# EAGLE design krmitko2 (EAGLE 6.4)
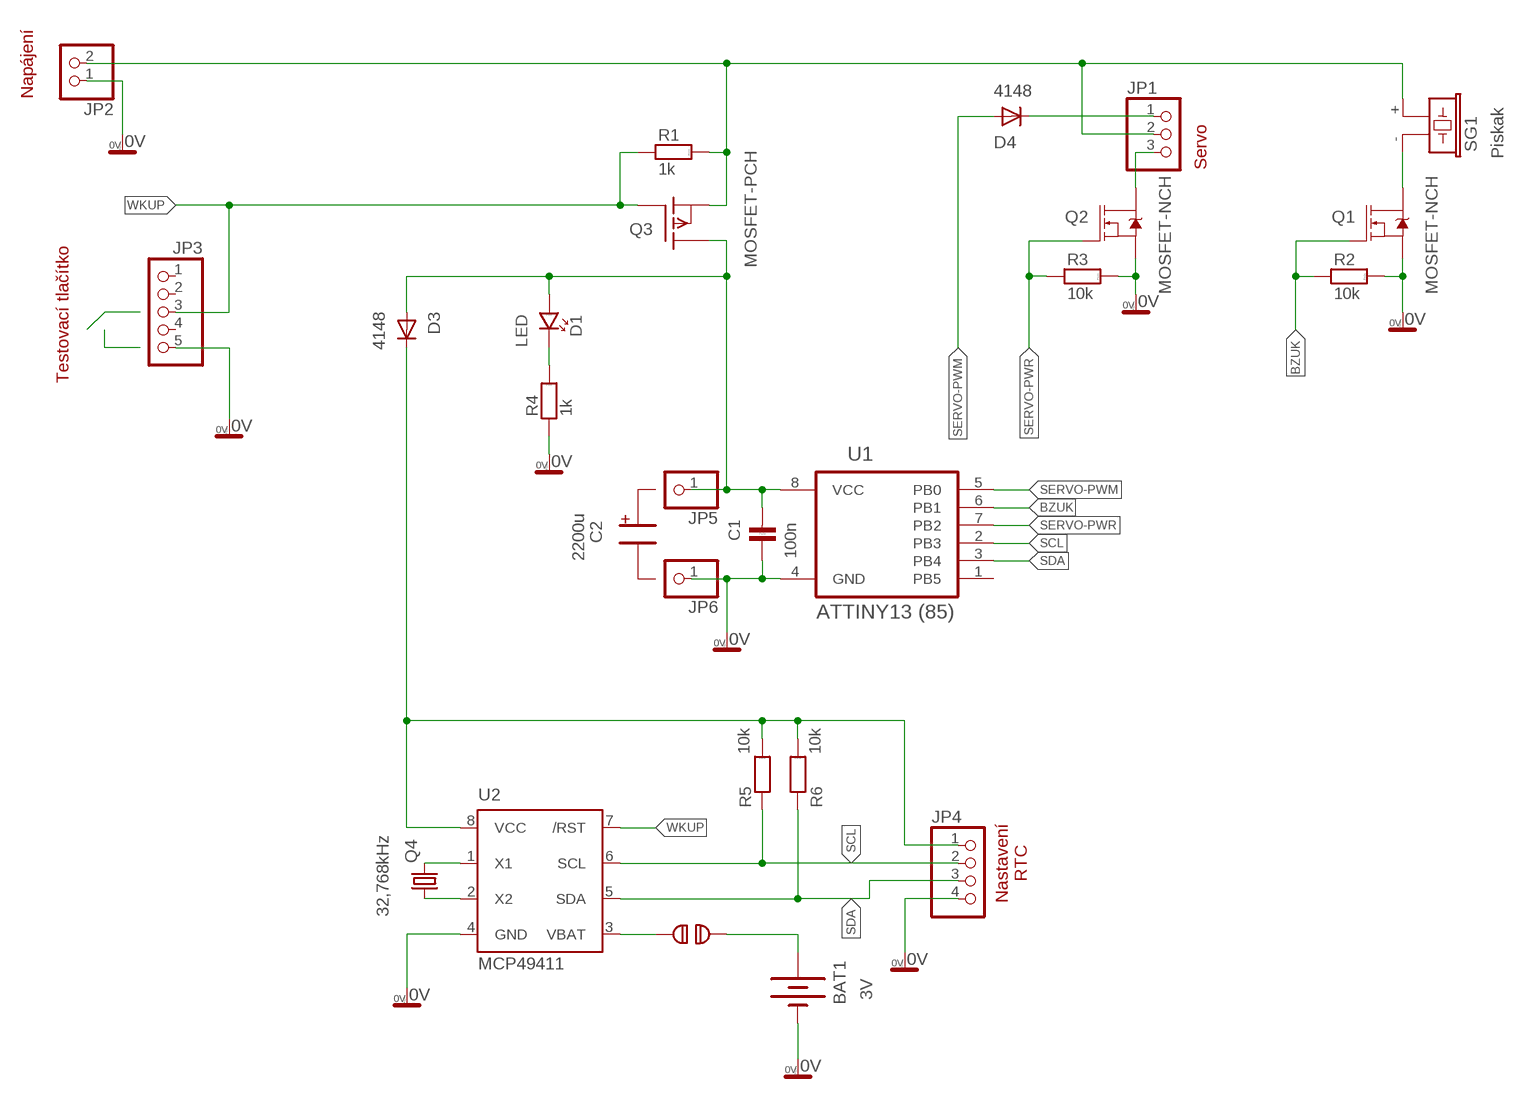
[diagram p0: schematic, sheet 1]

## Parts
BAT1  3V  BATTERY20PTH2  [BATTERY]
C1  100n  C-KER_0805  [0805]
D1  LED  LED_3  [LED_3]
D3  4148  CGRM4001-G  [SOD-123_MINI-SMA]
D4  4148  CGRM4001-G  [SOD-123_MINI-SMA]
JP1  PINHD-1X3  [1X03]
JP2  PINHD-1X2  [1X02]
JP3  PINHD-1X5  [1X05]
JP4  PINHD-1X4  [1X04]
JP5  PINHD-1X1  [1X01]
JP6  PINHD-1X1  [1X01]
Q1  MOSFET-NCH  [UNIFET]
Q2  MOSFET-NCH  [UNIFET]
Q3  MOSFET-PCH  LP0701N3  [TO-92]
Q4  32,768kHz  CRYSTALTC26H  [TC26H]
R1  1k  R_0805  [0805]
R2  10k  R_0805  [0805]
R3  10k  R_0805  [0805]
R4  1k  R_0805  [0805]
R5  10k  R_0805  [0805]
R6  10k  R_0805  [0805]
SG1  Piskak  F/CM12P  [F/CM12P]
U1  ATTINY13 (85)  ATTINY85-20PU  [DIP254P762X533-8]
U2  MCP49411  DS1672  [SOIC8]
U$1  SOLDERJUMPER  [SJ_2S-NO]

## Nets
0V: BAT1.- C1.1 JP2.1 JP3.5 JP4.4 JP6.1 Q1.S Q1.S2(S) Q2.S Q2.S2(S) R2.2 R3.2 R4.1 U1.4(GND) U2.4(GND)
BZUK: Q1.G R2.1 U1.6(PB1)
N$1: C1.2 D1.A D3.A JP5.1 Q3.3(D) U1.8(VCC)
N$2: BAT1.+ U$1.2
N$3: JP1.2 JP2.2 Q3.1(S) R1.2 SG1.+
N$4: Q1.D SG1.-
N$5: U2.3(VBAT) U$1.1
N$7: JP1.3 Q2.D
N$8: D4.C JP1.1
N$11: D1.K R4.2
N$14: Q4.2 U2.1(X1)
N$15: Q4.1 U2.2(X2)
SCL: JP4.2 R5.1 U1.2(PB3) U2.6(SCL)
SDA: JP4.3 R6.1 U1.3(PB4) U2.5(SDA)
SERVO-PWM: D4.A U1.5(PB0)
SERVO-PWR: Q2.G R3.1 U1.7(PB2)
VCC-RTC: D3.C JP4.1 R5.2 R6.2 U2.8(VCC)
WKUP: JP3.3 Q3.2(G) R1.1 U2.7(/RST)
Unconnected: JP3.1 JP3.2 JP3.4 U1.1(PB5)

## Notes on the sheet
- Napájení
- Servo
- Testovací tlačítko
- +
- C2
- 2200u
- Nastavení
  RTC

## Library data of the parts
BAT1 = bat2032-3pin:BATTERY: Battery Holders
C1 = #PaJa_31:C-KER: Kondenzator - keramicky
D1 = #PaJa_30:LED: LED - jednobarevna
D3 D4 = diode:CGRM400*-G: Molded plasitc,JEDEC SOD-123/Mini SMA
JP1 = uprava-pinhead:PINHD-1X3: PIN HEADER
JP2 = uprava-pinhead:PINHD-1X2: PIN HEADER
JP3 = pinhead:PINHD-1X5: PIN HEADER
JP4 = pinhead:PINHD-1X4: PIN HEADER
JP5 JP6 = pinhead:PINHD-1X1: PIN HEADER
Q1 Q2 = unifet4:MOSFET-NCH: Univerzalni prostor pro osazeni libovolne orientovaneho N-Fetu
Q3 = transistor-fet:LP0701N3: P-Channel Enhancement MOSFET -16,5V; -1,25A; 1,5Ohm
Q4 = adafruit:CRYSTAL: CRYSTAL; OC_FARNELL: unknown; OC_NEWARK: unknown
R1-R6 = #PaJa_31:R: Rezistor
SG1 = buzzer:F/CM12P: BUZZER; OC_FARNELL: unknown; OC_NEWARK: unknown
U1 = Atmel_By_element14_Batch_1-00:ATTINY85-20PU: 8-bit Microcontroller with In-System Programmable Flash; MPN: ATTINY85-20PU; OC_FARNELL: 1455162; OC_NEWARK: 58M3796; PACKAGE: PDIP-8; SUPPLIER: Atmel
U2 = ds1672:DS1672: RTC - I2C 32-bitový binární sekundový čítač
U$1 = solderjump:SOLDERJUMPER: Pájecí propojka

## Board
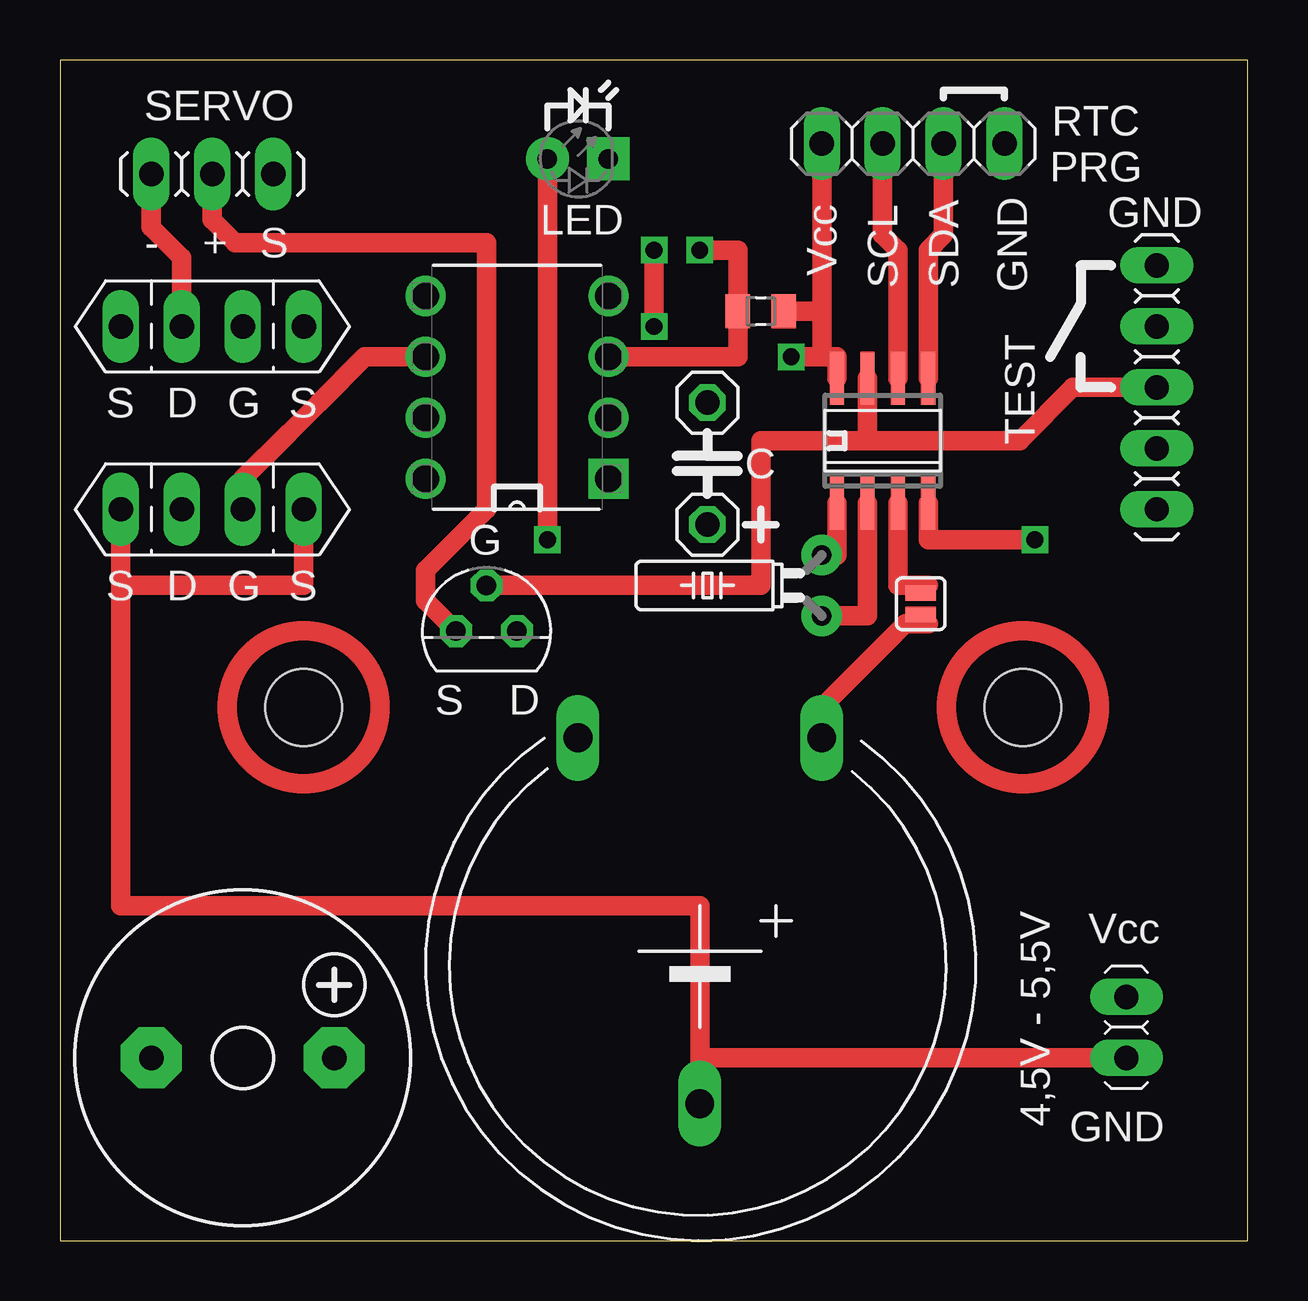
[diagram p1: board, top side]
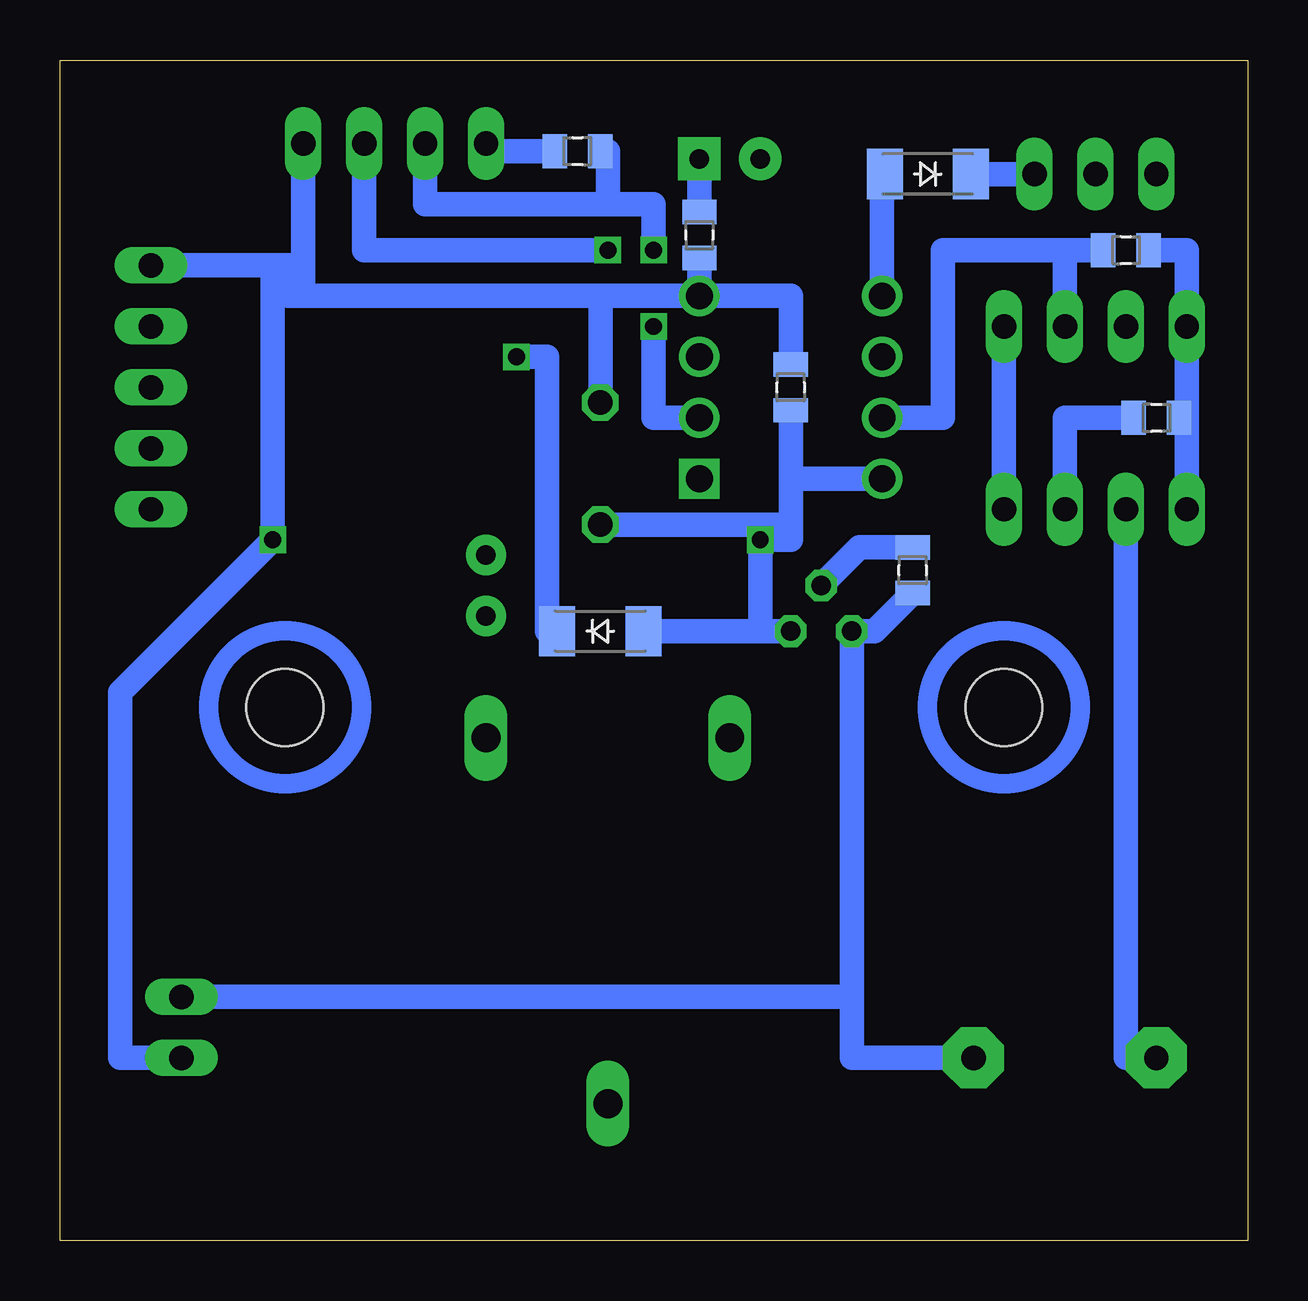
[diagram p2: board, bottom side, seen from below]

Size 49.51 x 49.2 mm. Coordinates in mm from the lower left corner, seen from the top.
Outline: 0,0 49.51,0 49.51,49.2 0,49.2 0,0
Copper layers (1*16): Top 0.035mm / dielectric 1.5mm / Bottom 0.035mm
Design rules "default": minimum track width 10mil, minimum drill 24mil, track to track 8mil, track to pad 8mil, pad to pad 8mil, via to via 8mil, smd to smd 8mil, copper to edge 40mil, drill to drill 8mil, minimum pad ring 10mil, minimum via ring 8mil, stop-mask expansion 4mil, vias tented up to drill 0mil, thermal gap 10mil
Holes 3.2 mm at 10.16,22.23 40.13,22.23

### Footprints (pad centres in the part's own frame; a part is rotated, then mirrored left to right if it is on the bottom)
BATTERY = drill 1.2 long: + 9.525,-5.08; +@1 9.525,5.08; - -5.715,0
0805 = smd 1.016 x 1.422: 1 -0.953,0; 2 0.953,0
LED_3 = drill 0.813 pad 1.778: A -1.27,0 | drill 0.813 pad 1.778 square: K 1.27,0
SOD-123_MINI-SMA = smd 1.5 x 2.1: A 1.8,0; C -1.8,0
1X03 = drill 1.016 long: 1 -2.54,0; 2 0,0; 3 2.54,0
1X02 = drill 1.016 long: 1 -1.27,0; 2 1.27,0
1X05 = drill 1.016 long: 1 -5.08,0; 2 -2.54,0; 3 0,0; 4 2.54,0; 5 5.08,0
1X04 = drill 1.016 long: 1 -3.81,0; 2 -1.27,0; 3 1.27,0; 4 3.81,0
1X01 = drill 1.016 octagon: 1 0,0
UNIFET = drill 1.016 long: D -1.27,0; G 1.27,0; S -3.81,0; S2 3.81,0
TO-92 = drill 0.813 octagon: 1 -1.27,0; 2 0,1.905; 3 1.27,0
TC26H = drill 0.813 pad 1.676: 1 -1.27,0; 2 1.27,0
F/CM12P = drill 1.016 pad 2.54 octagon: + 3.81,0; - -3.81,0
DIP254P762X533-8 = drill 1.118 square: 1 -7.62,7.62 | drill 1.118: 2 -7.62,5.08; 3 -7.62,2.54; 4 -7.62,0; 5 0,0; 6 0,2.54; 7 0,5.08; 8 0,7.62
SOIC8 = smd 0.6 x 2.2: 1 -1.905,-2.6; 2 -0.635,-2.6; 3 0.635,-2.6; 4 1.905,-2.6; 5 1.905,2.6; 6 0.635,2.6; 7 -0.635,2.6; 8 -1.905,2.6
SJ_2S-NO = smd 0.635 x 1.27: 1 0,0; 2 0.889,0

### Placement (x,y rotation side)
BAT1  26.67,11.43 90 top
C1  19.05,35.56 270 bottom
D1  21.59,45.09 0 top
D3  26.99,25.4 0 bottom
D4  13.34,44.45 180 bottom
JP1  6.35,44.45 180 top
JP2  44.45,8.89 90 top
JP3  45.72,35.56 90 top
JP4  35.56,45.72 0 top
JP5  26.99,29.84 0 top
JP6  26.99,34.92 0 top
Q1  6.35,30.48 0 top
Q2  6.35,38.1 0 top
Q3  17.78,25.4 0 top
Q4  31.75,27.3 90 top
R1  13.97,27.94 270 bottom
R2  3.81,34.29 0 bottom
R3  5.08,41.27 0 bottom
R4  22.86,41.91 90 bottom
R5  27.94,45.4 180 bottom
R6  29.21,38.73 0 top
SG1  7.62,7.62 0 top
U1  15.24,39.37 180 top
U2  34.29,33.34 0 top
U$1  35.88,26.99 270 top

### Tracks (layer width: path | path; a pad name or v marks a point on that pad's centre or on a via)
0V  (via drill 0.7)
  Top 0.813: JP2.1 26.67,7.62 BAT1.- 26.67,13.97 2.54,13.97 2.54,27.3 | U2.4 36.2,29.21 v40.64,29.21 | 2.54,27.3 Q1.S | Q1.S2 10.16,27.3 2.54,27.3
  Bottom 0.813: JP4.4 39.37,40.64 | R2.2 2.54,34.29
  Bottom 1.016: 40.64,40.64 v40.64,29.21 46.99,22.86 46.99,7.62 JP2.1 | 40.64,40.64 JP3.5 | 39.37,40.64 40.64,40.64 | R3.2 2.54,41.27 Q2.S 2.54,34.29 Q1.S | U1.4 19.05,39.37 C1.1 | Q2.S2 Q1.S2 | U1.4 R4.1 | U1.4 26.99,39.37 | 26.99,39.37 38.42,39.37 39.37,39.37 | 39.37,39.37 JP4.4 | JP6.1 26.99,39.37 | 39.37,39.37 40.01,39.37 40.01,40.01
BZUK
  Top 0.813: U1.6 12.7,36.83 10.79,34.92 9.53,33.66 7.62,31.75 Q1.G
  Bottom 1.016: R2.1 7.62,34.29 Q1.G
N$1  (via drill 0.7)
  Top 0.813: D1.A v20.32,29.21
  Bottom 0.813: Q3.3 20.32,25.4
  Bottom 1.016: U1.8 19.05,31.75 | 19.05,31.75 C1.2 | D3.A Q3.3 | 19.05,31.75 19.05,29.84 | JP5.1 19.05,29.84 | 19.05,29.84 19.05,29.21 v20.32,29.21 20.32,25.4
N$2
  Top 0.305: 36.2,25.72 36.2,25.78 U$1.2
  Top 0.813: BAT1.+ 31.75,22.23 35.24,25.72 36.2,25.72
N$3
  Top 0.813: Q3.1 15.24,26.67 15.24,27.94 17.78,30.48 17.78,41.59 7.3,41.59 6.35,42.55 JP1.2
  Bottom 1.016: JP2.2 16.51,10.16 | 16.51,10.16 Q3.1 15.56,25.4 R1.2 | SG1.+ 16.51,7.62 16.51,10.16
N$4
  Bottom 1.016: Q1.D 5.08,7.62 SG1.-
N$5
  Top 0.305: 36.2,27.3 36.2,26.99 U$1.1
  Top 0.813: U2.3 34.92,27.3 36.2,27.3
N$7
  Top 0.813: JP1.3 3.81,42.23 5.08,40.96 Q2.D
N$8
  Bottom 1.016: JP1.1 D4.C
N$11
  Bottom 1.016: D1.K R4.2
N$14
  Top 0.813: U2.1 32.38,28.57 Q4.2
N$15
  Top 0.813: U2.2 33.66,26.04 Q4.1
SCL  (via drill 0.7)
  Top 0.813: U2.6 34.92,41.27 34.29,41.91 JP4.2 | v24.77,41.27 v24.77,38.1
  Bottom 1.016: JP4.2 34.29,43.18 26.67,43.18 | 26.67,43.18 24.77,43.18 v24.77,41.27 | v24.77,38.1 24.77,34.29 U1.2 | R5.1 26.67,45.4 26.67,43.18
SDA  (via drill 0.7)
  Top 0.813: U2.5 36.2,41.27 36.83,41.91 JP4.3 | U1.3 28.26,36.83 R6.1 28.26,41.27 v26.67,41.27
  Bottom 1.016: JP4.3 36.83,41.27 v26.67,41.27
SERVO-PWM
  Bottom 0.813: 15.24,44.34 D4.A
  Bottom 1.016: U1.5 15.24,44.34
SERVO-PWR
  Bottom 1.016: R3.1 7.62,41.27 | Q2.G 7.62,41.27 | 7.62,41.27 12.7,41.27 12.7,34.29 U1.7
VCC-RTC  (via drill 0.7)
  Top 0.813: v30.48,36.83 31.75,36.83 | JP4.1 31.75,38.73 | 31.75,38.73 R6.2 | 31.75,36.83 32.38,36.83 U2.8 | 31.75,36.83 31.75,38.73
  Bottom 0.813: 31.75,45.4 JP4.1
  Bottom 1.016: v30.48,36.83 29.21,36.83 29.21,25.4 D3.C | R5.2 31.75,45.4
WKUP
  Top 0.813: JP3.3 42.23,35.56 40.01,33.34 33.66,33.34 | 33.66,33.34 U2.7 | Q3.2 29.21,27.3 29.21,33.34 33.66,33.34
  Bottom 1.016: Q3.2 16.19,28.89 R1.1
(copper drawn outside any net)
  shapes: Bottom circle x2, Top circle x2

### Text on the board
tPlace: SERVO | RTC / PRG | LED | Vcc | GND | GND | - | + | S | SCL | SDA | TEST | C | G | S | D | Vcc | 4,5V - 5,5V | GND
